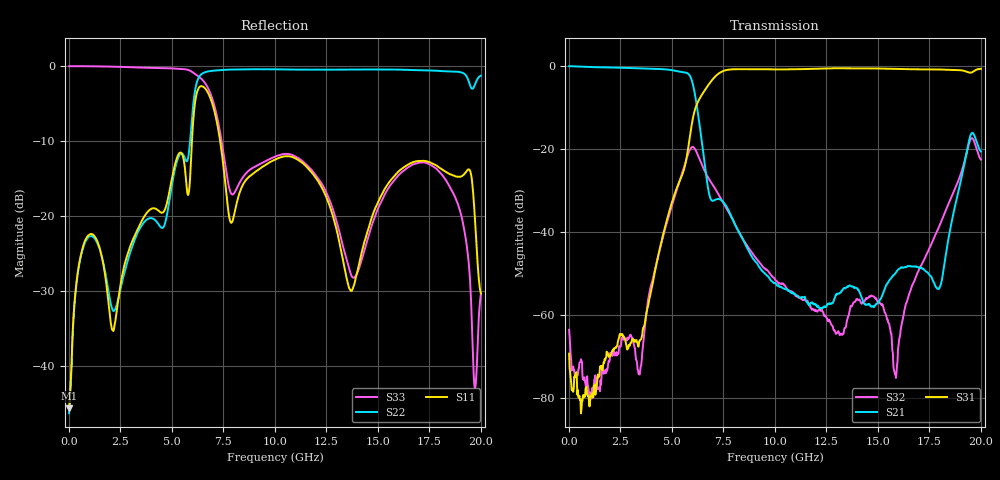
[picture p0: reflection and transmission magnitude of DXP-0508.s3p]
! MARKI MICROWAVE INC.
! Email:  info@markimicrowave.com  Phone:  408-778-4200
! Model Number:  DPX-0508  Date:  02/12
! Filename:		DPX-0508.S3P  Version: 1.0
! Description:  3-port S-parameter data for Diplexer DPX-0508
! Frequency Range: 	10 MHz to 20 GHz
! Port Configuration:	PORT 1: COMMON, PORT 2: LOW PASS, PORT 3: HIGH PASS
! S3P File: Measurements: Mag<S11> Ang<S11> Mag<S12> Ang<S12> Mag<S13> Ang<S13>! row 1
!  Mag<S21> Ang<S21> Mag<S22> Ang<S22> Mag<S23> Ang<S23>! row 2
!  Mag<S31> Ang<S31> Mag<S32> Ang<S32> Mag<S33> Ang<S33>! row 3
# Hz S  dB  R 50
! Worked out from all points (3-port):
!   801 points, 10 MHz to 20 GHz, reference 50 ohm
!   strongest paths, dB at 10 MHz, 5.008 GHz, 10.01 GHz, 15 GHz, 20 GHz:
!     S31: -69.4, -32.8, -0.8, -0.6, -0.7
!     S21: 0.0, -1.0, -52.3, -57.1, -20.6
!     S32: -63.6, -33.5, -51.4, -56.9, -22.5
!   lowest |S11| = -45.7 dB at 10 MHz (marker M1), VSWR 1.01, Z = 50.4 + j0.357 ohm
!   |S11| at or under -10 dB: start of sweep to 5.974 GHz; 7.342 GHz to end of sweep
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1e7  -45.73 43.2  -0.02 -5.4  -70.76 -1.9
     -0.02 -5.4  -46.38 18.7  -64.95 -145.4
     -69.35 -115.1  -63.62 21.7  0.00 -2.4
1.30935e9  -22.99 104.7  -0.27 -178.5  -72.84 -129.2
           -0.27 -178.4  -23.27 81.9  -75.74 51.9
           -78.31 -174.5  -78.31 -53.1  -0.02 -83.1
2.733638e9  -26.19 86.6  -0.44 -15.6  -64.99 104.3
            -0.43 -15.5  -27.18 64.6  -64.84 -126.3
            -65.99 111.4  -65.69 -127.2  -0.10 -175.2
5.982012e9  -9.56 -11.8  -3.73 142.7  -13.54 52.4
            -3.71 142.8  -6.70 85.8  -19.50 -162.2
            -13.56 52.5  -19.52 -162.1  -0.76 -53.9
7.256375e9  -8.55 65.6  -32.07 27.3  -1.83 -149.8
            -32.05 27.5  -0.53 -93.2  -30.87 -62.8
            -1.84 -149.6  -30.89 -62.8  -7.59 -171.4
1.0005e10  -12.48 -103.3  -52.55 174.4  -0.78 -75.1
           -52.27 173.3  -0.41 47.8  -51.14 -13.1
           -0.80 -74.8  -51.44 -11.5  -12.09 134.6
1.315342e10  -23.80 -32.1  -54.76 -21.0  -0.51 39.5
             -54.70 -22.1  -0.45 177.4  -64.75 110.1
             -0.51 39.7  -64.92 115.0  -22.36 -57.8
1.585208e10  -14.51 -26.8  -49.62 122.8  -0.68 -155.6
             -49.94 123.9  -0.45 1.2  -76.82 139.7
             -0.69 -155.5  -74.08 59.8  -15.03 -98.8
1.76012e10  -12.94 -155.7  -51.11 -83.8  -0.81 83.1
            -50.86 -82.6  -0.57 -108.7  -42.79 174.8
            -0.80 83.3  -42.89 174.5  -13.26 147.2
2e10  -30.36 86.9  -20.61 77.7  -0.66 -77.6
      -20.61 77.6  -1.25 114.2  -22.52 154.8
      -0.66 -77.1  -22.54 155.2  -30.38 -104.7
